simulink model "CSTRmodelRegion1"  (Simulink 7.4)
settings: Solver=ode15s  StartTime=0.0  StopTime=500  RelTol=1e-3
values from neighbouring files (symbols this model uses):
  cain = 2    [runDynSim321.m]    (also in sf_CSTR.m = cInVec(1))
  cbin = 1.5    [runDynSim321.m]    (also in sf_CSTR.m = cInVec(2))
undefined symbols (not defined in the file or in its folder): clamping, Floor, Ideal, internal, PI, sigbuilder_block
libraries: simulink_extras x2

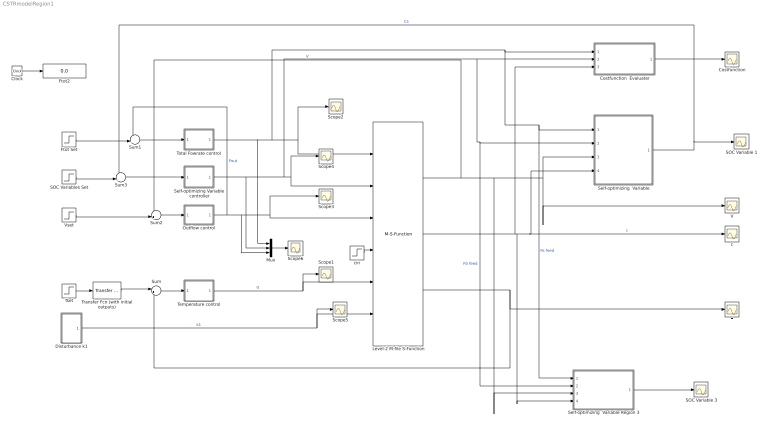
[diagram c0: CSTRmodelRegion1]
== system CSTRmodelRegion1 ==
  Clock : Clock
  Costfunction : Scope
  Costfunction  Evaluater : Subsystem
  Disturbance k1 : Subsystem
  Ftot Set : Step  Time=0  Before=22  After=22  SampleTime=0
  Ftot2 : Display
  Level-2 M-file S-Function : M-S-Function  FunctionName=sf_CSTR
  Mux : Mux  Inputs=3
  Outflow control : Subsystem  AncestorBlock=simulink/Continuous/PID Controller  DialogController=pidpack.PIDConfig.pidDDGCreate  DialogControllerArgs=DataTag2  mask(PID 1dof){Controller=PI, TimeDomain=Continuous-time, SampleTime=1, IntegratorMethod=Forward Euler, FilterMethod=Forward Euler, Form=Ideal, P=-5, I=0.8, D=0, N=100, InitialConditionSource=internal, InitialConditionForIntegrator=0, InitialConditionForFilter=0, ExternalReset=none, IgnoreLimit=off, ZeroCross=on, LimitOutput=off, UpperSaturationLimit=inf, LowerSaturationLimit=-inf, LinearizeAsGain=off, AntiWindupMode=none, Kb=1, TrackingMode=off, Kt=1, RndMeth=Floor, SaturateOnIntegerOverflow=off, LockScale=off, PParamMin=[], PParamMax=[], PParamDataTypeStr=Inherit: Inherit via internal rule, IParamMin=[], IParamMax=[], IParamDataTypeStr=Inherit: Inherit via internal rule, DParamMin=[], DParamMax=[], DParamDataTypeStr=Inherit: Inherit via internal rule, NParamMin=[], NParamMax=[], NParamDataTypeStr=Inherit: Inherit via internal rule, KbParamMin=[], KbParamMax=[], KbParamDataTypeStr=Inherit: Inherit via internal rule, KtParamMin=[], KtParamMax=[], KtParamDataTypeStr=Inherit: Inherit via internal rule, POutMin=[], POutMax=[], POutDataTypeStr=Inherit: Inherit via internal rule, IOutMin=[], IOutMax=[], IOutDataTypeStr=Inherit: Inherit via internal rule, DOutMin=[], DOutMax=[], DOutDataTypeStr=Inherit: Inherit via internal rule, NOutMin=[], NOutMax=[], NOutDataTypeStr=Inherit: Inherit via internal rule, KbOutMin=[], KbOutMax=[], KbOutDataTypeStr=Inherit: Inherit via internal rule, KtOutMin=[], KtOutMax=[], KtOutDataTypeStr=Inherit: Inherit via internal rule, IntegratorOutMin=[], IntegratorOutMax=[], IntegratorOutDataTypeStr=Inherit: Inherit via internal rule, FilterOutMin=[], FilterOutMax=[], FilterOutDataTypeStr=Inherit: Inherit via internal rule, SumOutMin=[], SumOutMax=[], SumOutDataTypeStr=Inherit: Inherit via internal rule, SumI1OutMin=[], SumI1OutMax=[], SumI1OutDataTypeStr=Inherit: Inherit via internal rule, SumI2OutMin=[], SumI2OutMax=[], SumI2OutDataTypeStr=Inherit: Inherit via internal rule, SumI3OutMin=[], SumI3OutMax=[], SumI3OutDataTypeStr=Inherit: Inherit via internal rule, SumDOutMin=[], SumDOutMax=[], SumDOutDataTypeStr=Inherit: Inherit via internal rule, SumAccumDataTypeStr=Inherit: Inherit via internal rule, SumI1AccumDataTypeStr=Inherit: Inherit via internal rule, SumI2AccumDataTypeStr=Inherit: Inherit via internal rule, SumI3AccumDataTypeStr=Inherit: Inherit via internal rule, SumDAccumDataTypeStr=Inherit: Inherit via internal rule, SaturationOutMin=[], SaturationOutMax=[], SaturationOutDataTypeStr=Inherit: Same as input, IntegratorContinuousStateAttributes='', IntegratorStateIdentifier=, IntegratorStateMustResolveToSignalObject=off, IntegratorRTWStateStorageClass=Auto, IntegratorRTWStateStorageTypeQualifier=, FilterContinuousStateAttributes='', FilterStateIdentifier=, FilterStateMustResolveToSignalObject=off, FilterRTWStateStorageClass=Auto, FilterRTWStateStorageTypeQualifier=}
      mask prompts: TimeDomain "Time-domain:"; SampleTime "Sample time (-1 for inherited):"; IntegratorMethod "Integrator method:"; FilterMethod "Filter method:"; Form "Controller form:"; P "Proportional (P):"; I "Integral (I):"; D "Derivative (D):"; N "Filter coefficient (N):"; InitialConditionSource "Source:"; InitialConditionForIntegrator "Integrator:"; InitialConditionForFilter "Filter:"; ExternalReset "External reset:"; IgnoreLimit "Ignore reset when linearizing"; ZeroCross "Enable zero-crossing detection"; LimitOutput "Limit output"; UpperSaturationLimit "Upper saturation limit:"; LowerSaturationLimit "Lower saturation limit:"; LinearizeAsGain "Ignore saturation when linearizing"; AntiWindupMode "Anti-windup method:"; Kb "Back-calculation coefficient (Kb):"; TrackingMode "Enable tracking mode"; Kt "Tracking coefficient (Kt):"; RndMeth "Integer rounding mode:"; SaturateOnIntegerOverflow "Saturate on integer overflow"; LockScale "Lock data type settings against changes by the fixed-point tools"; PParamMin "P parameter minimum:"; PParamMax "P parameter maximum:"; PParamDataTypeStr "P parameter:"; IParamMin "I parameter minimum:"; IParamMax "I parameter maximum:"; IParamDataTypeStr "I parameter:"; DParamMin "D parameter minimum:"; DParamMax "D parameter maximum:"; DParamDataTypeStr "D parameter:"; NParamMin "N parameter minimum:"; NParamMax "N parameter maximum:"; NParamDataTypeStr "N parameter:"; KbParamMin "Kb parameter minimum:"; KbParamMax "Kb parameter maximum:"; KbParamDataTypeStr "Kb parameter:"; KtParamMin "Kt parameter minimum:"; KtParamMax "Kt parameter maximum:"; KtParamDataTypeStr "Kt parameter:"; POutMin "P product output minimum:"; POutMax "P product output maximum:"; POutDataTypeStr "P product output:"; IOutMin "I product output minimum:"; IOutMax "I product output maximum:"; IOutDataTypeStr "I product output:"; DOutMin "D product output minimum:"; DOutMax "D product output maximum:"; DOutDataTypeStr "D product output:"; NOutMin "N product output minimum:"; NOutMax "N product output maximum:"; NOutDataTypeStr "N product output:"; KbOutMin "Kb product output minimum:"; KbOutMax "Kb product output maximum:"; KbOutDataTypeStr "Kb product output:"; KtOutMin "Kt product output minimum:"; KtOutMax "Kt product output maximum:"; KtOutDataTypeStr "Kt product output:"; IntegratorOutMin "Integrator output minimum:"; IntegratorOutMax "Integrator output maximum:"; IntegratorOutDataTypeStr "Integrator output:"; FilterOutMin "Filter output minimum:"; FilterOutMax "Filter output maximum:"; FilterOutDataTypeStr "Filter output:"; SumOutMin "Sum output minimum:"; SumOutMax "Sum output maximum:"; SumOutDataTypeStr "Sum output:"; SumI1OutMin "SumI1 output minimum:"; SumI1OutMax "SumI1 output maximum:"; SumI1OutDataTypeStr "SumI1 output:"; SumI2OutMin "SumI2 output minimum:"; SumI2OutMax "SumI2 output maximum:"; SumI2OutDataTypeStr "SumI2 output:"; SumI3OutMin "SumI3 output minimum:"; SumI3OutMax "SumI3 output maximum:"; SumI3OutDataTypeStr "SumI3 output:"; SumDOutMin "SumD output minimum:"; SumDOutMax "SumD output maximum:"; SumDOutDataTypeStr "SumD output:"; SumAccumDataTypeStr "Accumulator of Sum:"; SumI1AccumDataTypeStr "Accumulator of SumI1:"; SumI2AccumDataTypeStr "Accumulator of SumI2:"; SumI3AccumDataTypeStr "Accumulator of SumI3:"; SumDAccumDataTypeStr "Accumulator of SumD:"; SaturationOutMin "Saturation output minimum:"; SaturationOutMax "Saturation output maximum:"; SaturationOutDataTypeStr "Saturation output:"; IntegratorContinuousStateAttributes "State name: (e.g., 'position')"; IntegratorStateIdentifier "State name:"; IntegratorStateMustResolveToSignalObject "State name must resolve to Simulink signal object"; IntegratorRTWStateStorageClass "Real-Time Workshop storage class:"; IntegratorRTWStateStorageTypeQualifier "Real-Time Workshop storage type qualifier:"; FilterContinuousStateAttributes "State name: (e.g., 'position')"; FilterStateIdentifier "State name:"; FilterStateMustResolveToSignalObject "State name must resolve to Simulink signal object"; FilterRTWStateStorageClass "Real-Time Workshop storage class:"; FilterRTWStateStorageTypeQualifier "Real-Time Workshop storage type qualifier:"
      mask help: This block implements continuous- and discrete-time PID control algorithms and includes advanced features such as anti-windup, external reset, and signal tracking. You can tune the PID gains automatically using the 'Tune...' button (requires Simulink Control Design).
      mask init:
      | [shiftx shifty satshiftx satshifty] = pidpack.PIDConfig.configPID(gcbh);
  SOC Variable 1 : Scope
  SOC Variable 3 : Scope
  SOC Variables Set : Step  Time=0  After=0  SampleTime=0
  Scope{1..6} (6 alike) : Scope
  Self-optimizing  Variable : Stateflow chart
  Self-optimizing  Variable Region 3 : Stateflow chart
  Self-optimizing Variable  controller : Subsystem  AncestorBlock=simulink/Continuous/PID Controller  DialogController=pidpack.PIDConfig.pidDDGCreate  DialogControllerArgs=DataTag3  mask(PID 1dof){Controller=PI, TimeDomain=Continuous-time, SampleTime=1, IntegratorMethod=Forward Euler, FilterMethod=Forward Euler, Form=Ideal, P=145, I=3, D=0, N=100, InitialConditionSource=internal, InitialConditionForIntegrator=0, InitialConditionForFilter=0, ExternalReset=none, IgnoreLimit=off, ZeroCross=on, LimitOutput=off, UpperSaturationLimit=1e6, LowerSaturationLimit=0, LinearizeAsGain=off, AntiWindupMode=none, Kb=1, TrackingMode=off, Kt=1, RndMeth=Floor, SaturateOnIntegerOverflow=off, LockScale=off, PParamMin=[], PParamMax=[], PParamDataTypeStr=Inherit: Inherit via internal rule, IParamMin=[], IParamMax=[], IParamDataTypeStr=Inherit: Inherit via internal rule, DParamMin=[], DParamMax=[], DParamDataTypeStr=Inherit: Inherit via internal rule, NParamMin=[], NParamMax=[], NParamDataTypeStr=Inherit: Inherit via internal rule, KbParamMin=[], KbParamMax=[], KbParamDataTypeStr=Inherit: Inherit via internal rule, KtParamMin=[], KtParamMax=[], KtParamDataTypeStr=Inherit: Inherit via internal rule, POutMin=[], POutMax=[], POutDataTypeStr=Inherit: Inherit via internal rule, IOutMin=[], IOutMax=[], IOutDataTypeStr=Inherit: Inherit via internal rule, DOutMin=[], DOutMax=[], DOutDataTypeStr=Inherit: Inherit via internal rule, NOutMin=[], NOutMax=[], NOutDataTypeStr=Inherit: Inherit via internal rule, KbOutMin=[], KbOutMax=[], KbOutDataTypeStr=Inherit: Inherit via internal rule, KtOutMin=[], KtOutMax=[], KtOutDataTypeStr=Inherit: Inherit via internal rule, IntegratorOutMin=[], IntegratorOutMax=[], IntegratorOutDataTypeStr=Inherit: Inherit via internal rule, FilterOutMin=[], FilterOutMax=[], FilterOutDataTypeStr=Inherit: Inherit via internal rule, SumOutMin=[], SumOutMax=[], SumOutDataTypeStr=Inherit: Inherit via internal rule, SumI1OutMin=[], SumI1OutMax=[], SumI1OutDataTypeStr=Inherit: Inherit via internal rule, SumI2OutMin=[], SumI2OutMax=[], SumI2OutDataTypeStr=Inherit: Inherit via internal rule, SumI3OutMin=[], SumI3OutMax=[], SumI3OutDataTypeStr=Inherit: Inherit via internal rule, SumDOutMin=[], SumDOutMax=[], SumDOutDataTypeStr=Inherit: Inherit via internal rule, SumAccumDataTypeStr=Inherit: Inherit via internal rule, SumI1AccumDataTypeStr=Inherit: Inherit via internal rule, SumI2AccumDataTypeStr=Inherit: Inherit via internal rule, SumI3AccumDataTypeStr=Inherit: Inherit via internal rule, SumDAccumDataTypeStr=Inherit: Inherit via internal rule, SaturationOutMin=[], SaturationOutMax=[], SaturationOutDataTypeStr=Inherit: Same as input, IntegratorContinuousStateAttributes='', IntegratorStateIdentifier=, IntegratorStateMustResolveToSignalObject=off, IntegratorRTWStateStorageClass=Auto, IntegratorRTWStateStorageTypeQualifier=, FilterContinuousStateAttributes='', FilterStateIdentifier=, FilterStateMustResolveToSignalObject=off, FilterRTWStateStorageClass=Auto, FilterRTWStateStorageTypeQualifier=}
      mask prompts: TimeDomain "Time-domain:"; SampleTime "Sample time (-1 for inherited):"; IntegratorMethod "Integrator method:"; FilterMethod "Filter method:"; Form "Controller form:"; P "Proportional (P):"; I "Integral (I):"; D "Derivative (D):"; N "Filter coefficient (N):"; InitialConditionSource "Source:"; InitialConditionForIntegrator "Integrator:"; InitialConditionForFilter "Filter:"; ExternalReset "External reset:"; IgnoreLimit "Ignore reset when linearizing"; ZeroCross "Enable zero-crossing detection"; LimitOutput "Limit output"; UpperSaturationLimit "Upper saturation limit:"; LowerSaturationLimit "Lower saturation limit:"; LinearizeAsGain "Ignore saturation when linearizing"; AntiWindupMode "Anti-windup method:"; Kb "Back-calculation coefficient (Kb):"; TrackingMode "Enable tracking mode"; Kt "Tracking coefficient (Kt):"; RndMeth "Integer rounding mode:"; SaturateOnIntegerOverflow "Saturate on integer overflow"; LockScale "Lock data type settings against changes by the fixed-point tools"; PParamMin "P parameter minimum:"; PParamMax "P parameter maximum:"; PParamDataTypeStr "P parameter:"; IParamMin "I parameter minimum:"; IParamMax "I parameter maximum:"; IParamDataTypeStr "I parameter:"; DParamMin "D parameter minimum:"; DParamMax "D parameter maximum:"; DParamDataTypeStr "D parameter:"; NParamMin "N parameter minimum:"; NParamMax "N parameter maximum:"; NParamDataTypeStr "N parameter:"; KbParamMin "Kb parameter minimum:"; KbParamMax "Kb parameter maximum:"; KbParamDataTypeStr "Kb parameter:"; KtParamMin "Kt parameter minimum:"; KtParamMax "Kt parameter maximum:"; KtParamDataTypeStr "Kt parameter:"; POutMin "P product output minimum:"; POutMax "P product output maximum:"; POutDataTypeStr "P product output:"; IOutMin "I product output minimum:"; IOutMax "I product output maximum:"; IOutDataTypeStr "I product output:"; DOutMin "D product output minimum:"; DOutMax "D product output maximum:"; DOutDataTypeStr "D product output:"; NOutMin "N product output minimum:"; NOutMax "N product output maximum:"; NOutDataTypeStr "N product output:"; KbOutMin "Kb product output minimum:"; KbOutMax "Kb product output maximum:"; KbOutDataTypeStr "Kb product output:"; KtOutMin "Kt product output minimum:"; KtOutMax "Kt product output maximum:"; KtOutDataTypeStr "Kt product output:"; IntegratorOutMin "Integrator output minimum:"; IntegratorOutMax "Integrator output maximum:"; IntegratorOutDataTypeStr "Integrator output:"; FilterOutMin "Filter output minimum:"; FilterOutMax "Filter output maximum:"; FilterOutDataTypeStr "Filter output:"; SumOutMin "Sum output minimum:"; SumOutMax "Sum output maximum:"; SumOutDataTypeStr "Sum output:"; SumI1OutMin "SumI1 output minimum:"; SumI1OutMax "SumI1 output maximum:"; SumI1OutDataTypeStr "SumI1 output:"; SumI2OutMin "SumI2 output minimum:"; SumI2OutMax "SumI2 output maximum:"; SumI2OutDataTypeStr "SumI2 output:"; SumI3OutMin "SumI3 output minimum:"; SumI3OutMax "SumI3 output maximum:"; SumI3OutDataTypeStr "SumI3 output:"; SumDOutMin "SumD output minimum:"; SumDOutMax "SumD output maximum:"; SumDOutDataTypeStr "SumD output:"; SumAccumDataTypeStr "Accumulator of Sum:"; SumI1AccumDataTypeStr "Accumulator of SumI1:"; SumI2AccumDataTypeStr "Accumulator of SumI2:"; SumI3AccumDataTypeStr "Accumulator of SumI3:"; SumDAccumDataTypeStr "Accumulator of SumD:"; SaturationOutMin "Saturation output minimum:"; SaturationOutMax "Saturation output maximum:"; SaturationOutDataTypeStr "Saturation output:"; IntegratorContinuousStateAttributes "State name: (e.g., 'position')"; IntegratorStateIdentifier "State name:"; IntegratorStateMustResolveToSignalObject "State name must resolve to Simulink signal object"; IntegratorRTWStateStorageClass "Real-Time Workshop storage class:"; IntegratorRTWStateStorageTypeQualifier "Real-Time Workshop storage type qualifier:"; FilterContinuousStateAttributes "State name: (e.g., 'position')"; FilterStateIdentifier "State name:"; FilterStateMustResolveToSignalObject "State name must resolve to Simulink signal object"; FilterRTWStateStorageClass "Real-Time Workshop storage class:"; FilterRTWStateStorageTypeQualifier "Real-Time Workshop storage type qualifier:"
      mask help: This block implements continuous- and discrete-time PID control algorithms and includes advanced features such as anti-windup, external reset, and signal tracking. You can tune the PID gains automatically using the 'Tune...' button (requires Simulink Control Design).
      mask init:
      | [shiftx shifty satshiftx satshifty] = pidpack.PIDConfig.configPID(gcbh);
  Sum : Sum  Inputs=|+-  OutDataType=fixdt(1, 16)  OutScaling=2^0
  Sum1 : Sum  Inputs=-+|  OutDataType=fixdt(1, 16)  OutScaling=2^0
  Sum2 : Sum  Inputs=-+|  OutDataType=fixdt(1, 16)  OutScaling=2^0
  Sum3 : Sum  Inputs=-+|  OutDataType=fixdt(1, 16)  OutScaling=2^0
  T : Scope
  Temperature control : Subsystem  AncestorBlock=simulink/Continuous/PID Controller  DialogController=pidpack.PIDConfig.pidDDGCreate  DialogControllerArgs=DataTag4  mask(PID 1dof){Controller=PI, TimeDomain=Continuous-time, SampleTime=1, IntegratorMethod=Forward Euler, FilterMethod=Forward Euler, Form=Ideal, P=-3521, I=2.4, D=0, N=100, InitialConditionSource=internal, InitialConditionForIntegrator=888, InitialConditionForFilter=0, ExternalReset=none, IgnoreLimit=off, ZeroCross=on, LimitOutput=on, UpperSaturationLimit=1e3, LowerSaturationLimit=0, LinearizeAsGain=off, AntiWindupMode=clamping, Kb=1, TrackingMode=off, Kt=1, RndMeth=Floor, SaturateOnIntegerOverflow=off, LockScale=off, PParamMin=[], PParamMax=[], PParamDataTypeStr=Inherit: Inherit via internal rule, IParamMin=[], IParamMax=[], IParamDataTypeStr=Inherit: Inherit via internal rule, DParamMin=[], DParamMax=[], DParamDataTypeStr=Inherit: Inherit via internal rule, NParamMin=[], NParamMax=[], NParamDataTypeStr=Inherit: Inherit via internal rule, KbParamMin=[], KbParamMax=[], KbParamDataTypeStr=Inherit: Inherit via internal rule, KtParamMin=[], KtParamMax=[], KtParamDataTypeStr=Inherit: Inherit via internal rule, POutMin=[], POutMax=[], POutDataTypeStr=Inherit: Inherit via internal rule, IOutMin=[], IOutMax=[], IOutDataTypeStr=Inherit: Inherit via internal rule, DOutMin=[], DOutMax=[], DOutDataTypeStr=Inherit: Inherit via internal rule, NOutMin=[], NOutMax=[], NOutDataTypeStr=Inherit: Inherit via internal rule, KbOutMin=[], KbOutMax=[], KbOutDataTypeStr=Inherit: Inherit via internal rule, KtOutMin=[], KtOutMax=[], KtOutDataTypeStr=Inherit: Inherit via internal rule, IntegratorOutMin=[], IntegratorOutMax=[], IntegratorOutDataTypeStr=Inherit: Inherit via internal rule, FilterOutMin=[], FilterOutMax=[], FilterOutDataTypeStr=Inherit: Inherit via internal rule, SumOutMin=[], SumOutMax=[], SumOutDataTypeStr=Inherit: Inherit via internal rule, SumI1OutMin=[], SumI1OutMax=[], SumI1OutDataTypeStr=Inherit: Inherit via internal rule, SumI2OutMin=[], SumI2OutMax=[], SumI2OutDataTypeStr=Inherit: Inherit via internal rule, SumI3OutMin=[], SumI3OutMax=[], SumI3OutDataTypeStr=Inherit: Inherit via internal rule, SumDOutMin=[], SumDOutMax=[], SumDOutDataTypeStr=Inherit: Inherit via internal rule, SumAccumDataTypeStr=Inherit: Inherit via internal rule, SumI1AccumDataTypeStr=Inherit: Inherit via internal rule, SumI2AccumDataTypeStr=Inherit: Inherit via internal rule, SumI3AccumDataTypeStr=Inherit: Inherit via internal rule, SumDAccumDataTypeStr=Inherit: Inherit via internal rule, SaturationOutMin=[], SaturationOutMax=[], SaturationOutDataTypeStr=Inherit: Same as input, IntegratorContinuousStateAttributes='', IntegratorStateIdentifier=, IntegratorStateMustResolveToSignalObject=off, IntegratorRTWStateStorageClass=Auto, IntegratorRTWStateStorageTypeQualifier=, FilterContinuousStateAttributes='', FilterStateIdentifier=, FilterStateMustResolveToSignalObject=off, FilterRTWStateStorageClass=Auto, FilterRTWStateStorageTypeQualifier=}
      mask prompts: TimeDomain "Time-domain:"; SampleTime "Sample time (-1 for inherited):"; IntegratorMethod "Integrator method:"; FilterMethod "Filter method:"; Form "Controller form:"; P "Proportional (P):"; I "Integral (I):"; D "Derivative (D):"; N "Filter coefficient (N):"; InitialConditionSource "Source:"; InitialConditionForIntegrator "Integrator:"; InitialConditionForFilter "Filter:"; ExternalReset "External reset:"; IgnoreLimit "Ignore reset when linearizing"; ZeroCross "Enable zero-crossing detection"; LimitOutput "Limit output"; UpperSaturationLimit "Upper saturation limit:"; LowerSaturationLimit "Lower saturation limit:"; LinearizeAsGain "Ignore saturation when linearizing"; AntiWindupMode "Anti-windup method:"; Kb "Back-calculation coefficient (Kb):"; TrackingMode "Enable tracking mode"; Kt "Tracking coefficient (Kt):"; RndMeth "Integer rounding mode:"; SaturateOnIntegerOverflow "Saturate on integer overflow"; LockScale "Lock data type settings against changes by the fixed-point tools"; PParamMin "P parameter minimum:"; PParamMax "P parameter maximum:"; PParamDataTypeStr "P parameter:"; IParamMin "I parameter minimum:"; IParamMax "I parameter maximum:"; IParamDataTypeStr "I parameter:"; DParamMin "D parameter minimum:"; DParamMax "D parameter maximum:"; DParamDataTypeStr "D parameter:"; NParamMin "N parameter minimum:"; NParamMax "N parameter maximum:"; NParamDataTypeStr "N parameter:"; KbParamMin "Kb parameter minimum:"; KbParamMax "Kb parameter maximum:"; KbParamDataTypeStr "Kb parameter:"; KtParamMin "Kt parameter minimum:"; KtParamMax "Kt parameter maximum:"; KtParamDataTypeStr "Kt parameter:"; POutMin "P product output minimum:"; POutMax "P product output maximum:"; POutDataTypeStr "P product output:"; IOutMin "I product output minimum:"; IOutMax "I product output maximum:"; IOutDataTypeStr "I product output:"; DOutMin "D product output minimum:"; DOutMax "D product output maximum:"; DOutDataTypeStr "D product output:"; NOutMin "N product output minimum:"; NOutMax "N product output maximum:"; NOutDataTypeStr "N product output:"; KbOutMin "Kb product output minimum:"; KbOutMax "Kb product output maximum:"; KbOutDataTypeStr "Kb product output:"; KtOutMin "Kt product output minimum:"; KtOutMax "Kt product output maximum:"; KtOutDataTypeStr "Kt product output:"; IntegratorOutMin "Integrator output minimum:"; IntegratorOutMax "Integrator output maximum:"; IntegratorOutDataTypeStr "Integrator output:"; FilterOutMin "Filter output minimum:"; FilterOutMax "Filter output maximum:"; FilterOutDataTypeStr "Filter output:"; SumOutMin "Sum output minimum:"; SumOutMax "Sum output maximum:"; SumOutDataTypeStr "Sum output:"; SumI1OutMin "SumI1 output minimum:"; SumI1OutMax "SumI1 output maximum:"; SumI1OutDataTypeStr "SumI1 output:"; SumI2OutMin "SumI2 output minimum:"; SumI2OutMax "SumI2 output maximum:"; SumI2OutDataTypeStr "SumI2 output:"; SumI3OutMin "SumI3 output minimum:"; SumI3OutMax "SumI3 output maximum:"; SumI3OutDataTypeStr "SumI3 output:"; SumDOutMin "SumD output minimum:"; SumDOutMax "SumD output maximum:"; SumDOutDataTypeStr "SumD output:"; SumAccumDataTypeStr "Accumulator of Sum:"; SumI1AccumDataTypeStr "Accumulator of SumI1:"; SumI2AccumDataTypeStr "Accumulator of SumI2:"; SumI3AccumDataTypeStr "Accumulator of SumI3:"; SumDAccumDataTypeStr "Accumulator of SumD:"; SaturationOutMin "Saturation output minimum:"; SaturationOutMax "Saturation output maximum:"; SaturationOutDataTypeStr "Saturation output:"; IntegratorContinuousStateAttributes "State name: (e.g., 'position')"; IntegratorStateIdentifier "State name:"; IntegratorStateMustResolveToSignalObject "State name must resolve to Simulink signal object"; IntegratorRTWStateStorageClass "Real-Time Workshop storage class:"; IntegratorRTWStateStorageTypeQualifier "Real-Time Workshop storage type qualifier:"; FilterContinuousStateAttributes "State name: (e.g., 'position')"; FilterStateIdentifier "State name:"; FilterStateMustResolveToSignalObject "State name must resolve to Simulink signal object"; FilterRTWStateStorageClass "Real-Time Workshop storage class:"; FilterRTWStateStorageTypeQualifier "Real-Time Workshop storage type qualifier:"
      mask help: This block implements continuous- and discrete-time PID control algorithms and includes advanced features such as anti-windup, external reset, and signal tracking. You can tune the PID gains automatically using the 'Tune...' button (requires Simulink Control Design).
      mask init:
      | [shiftx shifty satshiftx satshifty] = pidpack.PIDConfig.configPID(gcbh);
  Total Fowrate control : Subsystem  AncestorBlock=simulink/Continuous/PID Controller  DialogController=pidpack.PIDConfig.pidDDGCreate  DialogControllerArgs=DataTag5  mask(PID 1dof){Controller=PI, TimeDomain=Continuous-time, SampleTime=1, IntegratorMethod=Forward Euler, FilterMethod=Forward Euler, Form=Ideal, P=0.58, I=0.35, D=0, N=100, InitialConditionSource=internal, InitialConditionForIntegrator=0, InitialConditionForFilter=0, ExternalReset=none, IgnoreLimit=off, ZeroCross=on, LimitOutput=off, UpperSaturationLimit=1e6, LowerSaturationLimit=0, LinearizeAsGain=off, AntiWindupMode=none, Kb=1, TrackingMode=off, Kt=1, RndMeth=Floor, SaturateOnIntegerOverflow=off, LockScale=off, PParamMin=[], PParamMax=[], PParamDataTypeStr=Inherit: Inherit via internal rule, IParamMin=[], IParamMax=[], IParamDataTypeStr=Inherit: Inherit via internal rule, DParamMin=[], DParamMax=[], DParamDataTypeStr=Inherit: Inherit via internal rule, NParamMin=[], NParamMax=[], NParamDataTypeStr=Inherit: Inherit via internal rule, KbParamMin=[], KbParamMax=[], KbParamDataTypeStr=Inherit: Inherit via internal rule, KtParamMin=[], KtParamMax=[], KtParamDataTypeStr=Inherit: Inherit via internal rule, POutMin=[], POutMax=[], POutDataTypeStr=Inherit: Inherit via internal rule, IOutMin=[], IOutMax=[], IOutDataTypeStr=Inherit: Inherit via internal rule, DOutMin=[], DOutMax=[], DOutDataTypeStr=Inherit: Inherit via internal rule, NOutMin=[], NOutMax=[], NOutDataTypeStr=Inherit: Inherit via internal rule, KbOutMin=[], KbOutMax=[], KbOutDataTypeStr=Inherit: Inherit via internal rule, KtOutMin=[], KtOutMax=[], KtOutDataTypeStr=Inherit: Inherit via internal rule, IntegratorOutMin=[], IntegratorOutMax=[], IntegratorOutDataTypeStr=Inherit: Inherit via internal rule, FilterOutMin=[], FilterOutMax=[], FilterOutDataTypeStr=Inherit: Inherit via internal rule, SumOutMin=[], SumOutMax=[], SumOutDataTypeStr=Inherit: Inherit via internal rule, SumI1OutMin=[], SumI1OutMax=[], SumI1OutDataTypeStr=Inherit: Inherit via internal rule, SumI2OutMin=[], SumI2OutMax=[], SumI2OutDataTypeStr=Inherit: Inherit via internal rule, SumI3OutMin=[], SumI3OutMax=[], SumI3OutDataTypeStr=Inherit: Inherit via internal rule, SumDOutMin=[], SumDOutMax=[], SumDOutDataTypeStr=Inherit: Inherit via internal rule, SumAccumDataTypeStr=Inherit: Inherit via internal rule, SumI1AccumDataTypeStr=Inherit: Inherit via internal rule, SumI2AccumDataTypeStr=Inherit: Inherit via internal rule, SumI3AccumDataTypeStr=Inherit: Inherit via internal rule, SumDAccumDataTypeStr=Inherit: Inherit via internal rule, SaturationOutMin=[], SaturationOutMax=[], SaturationOutDataTypeStr=Inherit: Same as input, IntegratorContinuousStateAttributes='', IntegratorStateIdentifier=, IntegratorStateMustResolveToSignalObject=off, IntegratorRTWStateStorageClass=Auto, IntegratorRTWStateStorageTypeQualifier=, FilterContinuousStateAttributes='', FilterStateIdentifier=, FilterStateMustResolveToSignalObject=off, FilterRTWStateStorageClass=Auto, FilterRTWStateStorageTypeQualifier=}
      mask prompts: TimeDomain "Time-domain:"; SampleTime "Sample time (-1 for inherited):"; IntegratorMethod "Integrator method:"; FilterMethod "Filter method:"; Form "Controller form:"; P "Proportional (P):"; I "Integral (I):"; D "Derivative (D):"; N "Filter coefficient (N):"; InitialConditionSource "Source:"; InitialConditionForIntegrator "Integrator:"; InitialConditionForFilter "Filter:"; ExternalReset "External reset:"; IgnoreLimit "Ignore reset when linearizing"; ZeroCross "Enable zero-crossing detection"; LimitOutput "Limit output"; UpperSaturationLimit "Upper saturation limit:"; LowerSaturationLimit "Lower saturation limit:"; LinearizeAsGain "Ignore saturation when linearizing"; AntiWindupMode "Anti-windup method:"; Kb "Back-calculation coefficient (Kb):"; TrackingMode "Enable tracking mode"; Kt "Tracking coefficient (Kt):"; RndMeth "Integer rounding mode:"; SaturateOnIntegerOverflow "Saturate on integer overflow"; LockScale "Lock data type settings against changes by the fixed-point tools"; PParamMin "P parameter minimum:"; PParamMax "P parameter maximum:"; PParamDataTypeStr "P parameter:"; IParamMin "I parameter minimum:"; IParamMax "I parameter maximum:"; IParamDataTypeStr "I parameter:"; DParamMin "D parameter minimum:"; DParamMax "D parameter maximum:"; DParamDataTypeStr "D parameter:"; NParamMin "N parameter minimum:"; NParamMax "N parameter maximum:"; NParamDataTypeStr "N parameter:"; KbParamMin "Kb parameter minimum:"; KbParamMax "Kb parameter maximum:"; KbParamDataTypeStr "Kb parameter:"; KtParamMin "Kt parameter minimum:"; KtParamMax "Kt parameter maximum:"; KtParamDataTypeStr "Kt parameter:"; POutMin "P product output minimum:"; POutMax "P product output maximum:"; POutDataTypeStr "P product output:"; IOutMin "I product output minimum:"; IOutMax "I product output maximum:"; IOutDataTypeStr "I product output:"; DOutMin "D product output minimum:"; DOutMax "D product output maximum:"; DOutDataTypeStr "D product output:"; NOutMin "N product output minimum:"; NOutMax "N product output maximum:"; NOutDataTypeStr "N product output:"; KbOutMin "Kb product output minimum:"; KbOutMax "Kb product output maximum:"; KbOutDataTypeStr "Kb product output:"; KtOutMin "Kt product output minimum:"; KtOutMax "Kt product output maximum:"; KtOutDataTypeStr "Kt product output:"; IntegratorOutMin "Integrator output minimum:"; IntegratorOutMax "Integrator output maximum:"; IntegratorOutDataTypeStr "Integrator output:"; FilterOutMin "Filter output minimum:"; FilterOutMax "Filter output maximum:"; FilterOutDataTypeStr "Filter output:"; SumOutMin "Sum output minimum:"; SumOutMax "Sum output maximum:"; SumOutDataTypeStr "Sum output:"; SumI1OutMin "SumI1 output minimum:"; SumI1OutMax "SumI1 output maximum:"; SumI1OutDataTypeStr "SumI1 output:"; SumI2OutMin "SumI2 output minimum:"; SumI2OutMax "SumI2 output maximum:"; SumI2OutDataTypeStr "SumI2 output:"; SumI3OutMin "SumI3 output minimum:"; SumI3OutMax "SumI3 output maximum:"; SumI3OutDataTypeStr "SumI3 output:"; SumDOutMin "SumD output minimum:"; SumDOutMax "SumD output maximum:"; SumDOutDataTypeStr "SumD output:"; SumAccumDataTypeStr "Accumulator of Sum:"; SumI1AccumDataTypeStr "Accumulator of SumI1:"; SumI2AccumDataTypeStr "Accumulator of SumI2:"; SumI3AccumDataTypeStr "Accumulator of SumI3:"; SumDAccumDataTypeStr "Accumulator of SumD:"; SaturationOutMin "Saturation output minimum:"; SaturationOutMax "Saturation output maximum:"; SaturationOutDataTypeStr "Saturation output:"; IntegratorContinuousStateAttributes "State name: (e.g., 'position')"; IntegratorStateIdentifier "State name:"; IntegratorStateMustResolveToSignalObject "State name must resolve to Simulink signal object"; IntegratorRTWStateStorageClass "Real-Time Workshop storage class:"; IntegratorRTWStateStorageTypeQualifier "Real-Time Workshop storage type qualifier:"; FilterContinuousStateAttributes "State name: (e.g., 'position')"; FilterStateIdentifier "State name:"; FilterStateMustResolveToSignalObject "State name must resolve to Simulink signal object"; FilterRTWStateStorageClass "Real-Time Workshop storage class:"; FilterRTWStateStorageTypeQualifier "Real-Time Workshop storage type qualifier:"
      mask help: This block implements continuous- and discrete-time PID control algorithms and includes advanced features such as anti-windup, external reset, and signal tracking. You can tune the PID gains automatically using the 'Tune...' button (requires Simulink Control Design).
      mask init:
      | [shiftx shifty satshiftx satshifty] = pidpack.PIDConfig.configPID(gcbh);
  Transfer Fcn (with initial outputs) : simulink_extras/Additional Linear/Transfer Fcn (with initial outputs)  SystemSampleTime=-1  N=[1]  D="[10  1]"  Y0=350  U0=0
  Tset : Step  Time=250  Before=350  After=350  SampleTime=0
  V : Scope
  Vset : Step  Time=0  Before=500  After=500  SampleTime=0
  c : Scope
  cin : Step  Time=0  Before=[cain cbin 0 0]  After=[cain cbin 0 0]  SampleTime=0
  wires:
  cin/1 -> Level-2 M-file S-Function/4
  Sum/1 -> Temperature control/1(u)
  Level-2 M-file S-Function/1 -> Sum2/1, Self-optimizing  Variable/3(V), V/1, Self-optimizing  Variable Region 3/3(V)  "V"
  Level-2 M-file S-Function/2 -> Costfunction  Evaluater/3(Concentrations), c/1, Self-optimizing  Variable/4(cVector), Self-optimizing  Variable Region 3/4(cVector)  "c"
  Level-2 M-file S-Function/3 -> T/1, Sum/2  "T"
  Tset/1 -> Transfer Fcn (with initial outputs)/1
  Vset/1 -> Sum2/2
  Sum2/1 -> Outflow control/1(u)
  Costfunction  Evaluater/1(Objective) -> Costfunction/1
  Outflow control/1(y) -> Sum1/1, Level-2 M-file S-Function/3, Scope3/1, Mux/3  "Fout"
  Temperature control/1(y) -> Level-2 M-file S-Function/5, Scope1/1  "q"
  Sum1/1 -> Total Fowrate control/1(u)
  Total Fowrate control/1(y) -> Level-2 M-file S-Function/1, Scope2/1, Costfunction  Evaluater/1(Fa), Self-optimizing  Variable/1(Fa), Self-optimizing  Variable Region 3/1(Fa), Mux/1  "Fa feed"
  Self-optimizing  Variable/1(cs) -> Sum3/1, SOC Variable 1/1  "Cs"
  SOC Variables Set/1 -> Sum3/2
  Sum3/1 -> Self-optimizing Variable  controller/1(u)
  Self-optimizing Variable  controller/1(y) -> Level-2 M-file S-Function/2, Scope4/1, Costfunction  Evaluater/2(Fb), Self-optimizing  Variable Region 3/2(Fb), Self-optimizing  Variable/2(Fb), Mux/2  "Fb feed"
  Ftot Set/1 -> Sum1/2
  Disturbance k1/1(Out1) -> Level-2 M-file S-Function/6, Scope5/1  "k1"
  Transfer Fcn (with initial outputs)/1 -> Sum/1
  Mux/1 -> Scope6/1
  Clock/1 -> Ftot2/1
  Self-optimizing  Variable Region 3/1(cs) -> SOC Variable 3/1

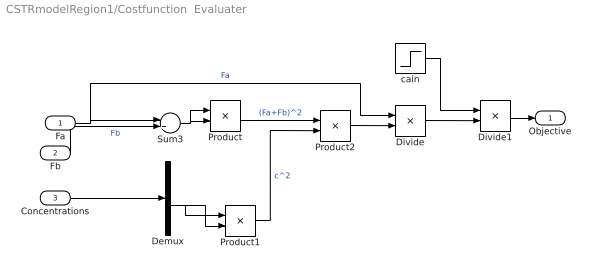
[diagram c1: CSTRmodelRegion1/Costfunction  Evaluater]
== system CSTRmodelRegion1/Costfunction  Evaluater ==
  Fa : Inport
  Fb : Inport  Port=2
  Concentrations : Inport  Port=3
  Demux : Demux
  Divide : Product  Inputs=/*  OutDataType=fixdt(1, 16)  OutScaling=2^-10
  Divide1 : Product  Inputs=/*  OutDataType=fixdt(1, 16)  OutScaling=2^-10
  Product : Product  OutDataType=fixdt(1, 16)  OutScaling=2^0
  Product1 : Product  OutDataType=fixdt(1, 16)  OutScaling=2^0
  Product2 : Product  OutDataType=fixdt(1, 16)  OutScaling=2^0
  Sum3 : Sum  Inputs=|++  OutDataType=fixdt(1, 16)  OutScaling=2^0
  cain : Step  Before=cain  After=cain  SampleTime=0
  Objective : Outport
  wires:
  Sum3/1 -> Product/1, Product/2
  Demux/3 -> Product1/2, Product1/1
  Product/1 -> Product2/1  "(Fa+Fb)^2"
  Product1/1 -> Product2/2  "c^2"
  Product2/1 -> Divide/2
  Divide/1 -> Divide1/2
  cain/1 -> Divide1/1
  Fa/1 -> Sum3/1, Divide/1  "Fa"
  Fb/1 -> Sum3/2  "Fb"
  Concentrations/1 -> Demux/1
  Divide1/1 -> Objective/1
  Demux/1 -> ?
  Demux/2 -> ?
  Demux/4 -> ?

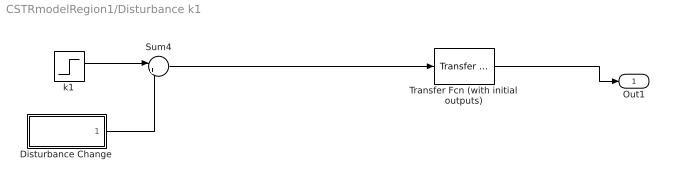
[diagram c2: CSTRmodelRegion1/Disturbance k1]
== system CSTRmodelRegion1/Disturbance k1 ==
  Disturbance Change : Subsystem  Tag=STV Subsys  LoadFcn=sigbuilder_block('load');  StartFcn=sigbuilder_block('start');  StopFcn=sigbuilder_block('stop');  ClipboardFcn=sigbuilder_block('clipboard');
  Sum4 : Sum  Inputs=|++  OutDataType=fixdt(1, 16)  OutScaling=2^0
  Transfer Fcn (with initial outputs) : simulink_extras/Additional Linear/Transfer Fcn (with initial outputs)  SystemSampleTime=-1  N=[1]  D="[2  1]"  Y0=0  U0=0
  k1 : Step  Time=200  Before=0.3  After=0.3  SampleTime=0
  Out1 : Outport
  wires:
  k1/1 -> Sum4/1
  Sum4/1 -> Transfer Fcn (with initial outputs)/1
  Transfer Fcn (with initial outputs)/1 -> Out1/1
  Disturbance Change/1(Signal 1) -> Sum4/2

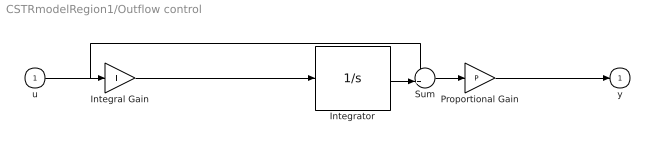
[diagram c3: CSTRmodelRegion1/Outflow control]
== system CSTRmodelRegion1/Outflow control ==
  u : Inport  OutDataType=OutDataTypeStr
  Integral Gain : Gain  DisableCoverage=on  Gain=I  ParamMin=IParamMin  ParamMax=IParamMax  ParameterDataTypeMode=Specify via dialog  ParameterDataType=IParamDataTypeStr  ParamDataTypeStr=IParamDataTypeStr  OutMin=IOutMin  OutMax=IOutMax  OutDataTypeMode=Specify via dialog  OutDataType=IOutDataTypeStr  OutDataTypeStr=IOutDataTypeStr
  Integrator : Integrator  DisableCoverage=on  InitialCondition=InitialConditionForIntegrator
  Proportional Gain : Gain  Gain=P  ParamMin=PParamMin  ParamMax=PParamMax  ParameterDataTypeMode=Specify via dialog  ParameterDataType=PParamDataTypeStr  ParamDataTypeStr=PParamDataTypeStr  OutMin=POutMin  OutMax=POutMax  OutDataTypeMode=Specify via dialog  OutDataType=POutDataTypeStr  OutDataTypeStr=POutDataTypeStr
  Sum : Sum  DisableCoverage=on  Inputs=++|  AccumDataTypeStr=SumAccumDataTypeStr  OutMin=SumOutMin  OutMax=SumOutMax  OutDataTypeMode=Specify via dialog  OutDataType=SumOutDataTypeStr  OutDataTypeStr=SumOutDataTypeStr
  y : Outport  OutDataType=OutDataTypeStr  InitialOutput=0
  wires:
  u/1 -> Sum/1, Integral Gain/1
  Proportional Gain/1 -> y/1
  Integral Gain/1 -> Integrator/1
  Integrator/1 -> Sum/2
  Sum/1 -> Proportional Gain/1

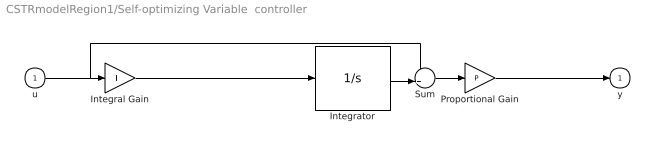
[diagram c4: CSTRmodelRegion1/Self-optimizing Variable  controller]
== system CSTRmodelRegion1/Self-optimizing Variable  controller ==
  u : Inport  OutDataType=OutDataTypeStr
  Integral Gain : Gain  DisableCoverage=on  Gain=I  ParamMin=IParamMin  ParamMax=IParamMax  ParameterDataTypeMode=Specify via dialog  ParameterDataType=IParamDataTypeStr  ParamDataTypeStr=IParamDataTypeStr  OutMin=IOutMin  OutMax=IOutMax  OutDataTypeMode=Specify via dialog  OutDataType=IOutDataTypeStr  OutDataTypeStr=IOutDataTypeStr
  Integrator : Integrator  DisableCoverage=on  InitialCondition=InitialConditionForIntegrator
  Proportional Gain : Gain  Gain=P  ParamMin=PParamMin  ParamMax=PParamMax  ParameterDataTypeMode=Specify via dialog  ParameterDataType=PParamDataTypeStr  ParamDataTypeStr=PParamDataTypeStr  OutMin=POutMin  OutMax=POutMax  OutDataTypeMode=Specify via dialog  OutDataType=POutDataTypeStr  OutDataTypeStr=POutDataTypeStr
  Sum : Sum  DisableCoverage=on  Inputs=++|  AccumDataTypeStr=SumAccumDataTypeStr  OutMin=SumOutMin  OutMax=SumOutMax  OutDataTypeMode=Specify via dialog  OutDataType=SumOutDataTypeStr  OutDataTypeStr=SumOutDataTypeStr
  y : Outport  OutDataType=OutDataTypeStr  InitialOutput=0
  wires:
  u/1 -> Sum/1, Integral Gain/1
  Proportional Gain/1 -> y/1
  Integral Gain/1 -> Integrator/1
  Integrator/1 -> Sum/2
  Sum/1 -> Proportional Gain/1

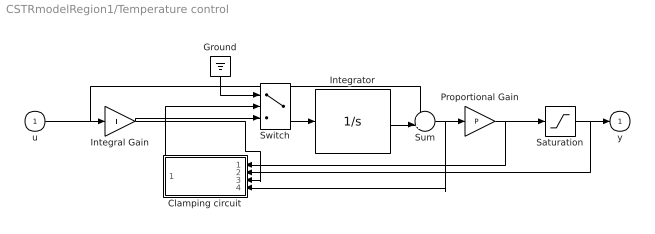
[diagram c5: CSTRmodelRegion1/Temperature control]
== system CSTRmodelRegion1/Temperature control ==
  u : Inport  OutDataType=OutDataTypeStr
  Clamping circuit : Subsystem
  Ground : Ground
  Integral Gain : Gain  DisableCoverage=on  Gain=I  ParamMin=IParamMin  ParamMax=IParamMax  ParameterDataTypeMode=Specify via dialog  ParameterDataType=IParamDataTypeStr  ParamDataTypeStr=IParamDataTypeStr  OutMin=IOutMin  OutMax=IOutMax  OutDataTypeMode=Specify via dialog  OutDataType=IOutDataTypeStr  OutDataTypeStr=IOutDataTypeStr
  Integrator : Integrator  DisableCoverage=on  InitialCondition=InitialConditionForIntegrator
  Proportional Gain : Gain  DisableCoverage=on  Gain=P  ParamMin=PParamMin  ParamMax=PParamMax  ParameterDataTypeMode=Specify via dialog  ParameterDataType=PParamDataTypeStr  ParamDataTypeStr=PParamDataTypeStr  OutMin=POutMin  OutMax=POutMax  OutDataTypeMode=Specify via dialog  OutDataType=POutDataTypeStr  OutDataTypeStr=POutDataTypeStr
  Saturation : Saturate  UpperLimit=UpperSaturationLimit  LowerLimit=LowerSaturationLimit  LinearizeAsGain=off  OutMin=SaturationOutMin  OutMax=SaturationOutMax  OutDataTypeMode=Specify via dialog  OutDataType=SaturationOutDataTypeStr  OutDataTypeStr=SaturationOutDataTypeStr
  Sum : Sum  DisableCoverage=on  Inputs=++|  AccumDataTypeStr=SumAccumDataTypeStr  OutMin=SumOutMin  OutMax=SumOutMax  OutDataTypeMode=Specify via dialog  OutDataType=SumOutDataTypeStr  OutDataTypeStr=SumOutDataTypeStr
  Switch : Switch  DisableCoverage=on  Criteria=u2 > Threshold
  y : Outport  OutDataType=OutDataTypeStr  InitialOutput=0
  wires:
  u/1 -> Sum/1, Integral Gain/1
  Integral Gain/1 -> Clamping circuit/3(preIntegrator), Switch/3
  Integrator/1 -> Sum/2
  Sum/1 -> Proportional Gain/1, Clamping circuit/4(preP)
  Saturation/1 -> y/1, Clamping circuit/2(postSat)
  Proportional Gain/1 -> Saturation/1, Clamping circuit/1(preSat)
  Ground/1 -> Switch/1
  Clamping circuit/1(Clamp) -> Switch/2
  Switch/1 -> Integrator/1

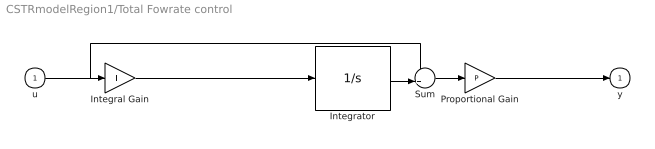
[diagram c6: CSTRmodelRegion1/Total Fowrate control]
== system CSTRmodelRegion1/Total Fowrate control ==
  u : Inport  OutDataType=OutDataTypeStr
  Integral Gain : Gain  DisableCoverage=on  Gain=I  ParamMin=IParamMin  ParamMax=IParamMax  ParameterDataTypeMode=Specify via dialog  ParameterDataType=IParamDataTypeStr  ParamDataTypeStr=IParamDataTypeStr  OutMin=IOutMin  OutMax=IOutMax  OutDataTypeMode=Specify via dialog  OutDataType=IOutDataTypeStr  OutDataTypeStr=IOutDataTypeStr
  Integrator : Integrator  DisableCoverage=on  InitialCondition=InitialConditionForIntegrator
  Proportional Gain : Gain  Gain=P  ParamMin=PParamMin  ParamMax=PParamMax  ParameterDataTypeMode=Specify via dialog  ParameterDataType=PParamDataTypeStr  ParamDataTypeStr=PParamDataTypeStr  OutMin=POutMin  OutMax=POutMax  OutDataTypeMode=Specify via dialog  OutDataType=POutDataTypeStr  OutDataTypeStr=POutDataTypeStr
  Sum : Sum  DisableCoverage=on  Inputs=++|  AccumDataTypeStr=SumAccumDataTypeStr  OutMin=SumOutMin  OutMax=SumOutMax  OutDataTypeMode=Specify via dialog  OutDataType=SumOutDataTypeStr  OutDataTypeStr=SumOutDataTypeStr
  y : Outport  OutDataType=OutDataTypeStr  InitialOutput=0
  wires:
  u/1 -> Sum/1, Integral Gain/1
  Proportional Gain/1 -> y/1
  Integral Gain/1 -> Integrator/1
  Integrator/1 -> Sum/2
  Sum/1 -> Proportional Gain/1

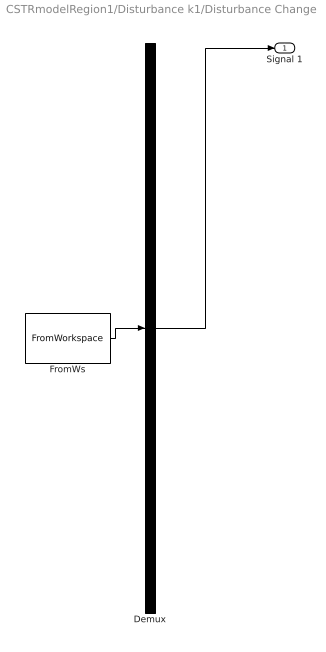
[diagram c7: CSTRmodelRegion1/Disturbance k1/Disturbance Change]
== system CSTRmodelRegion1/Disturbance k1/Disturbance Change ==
  Demux : Demux  Tag=STV Demux  Outputs=1
  FromWs : FromWorkspace  Tag=STV FromWs  VariableName=tuvar  SampleTime=0  SigBuilderData=DataTag0  VnvData=DataTag1
  Signal 1 : Outport  Tag=STV Outport  OutDataType=fixdt(1, 16)  OutScaling=2^0
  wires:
  FromWs/1 -> Demux/1
  Demux/1 -> Signal 1/1

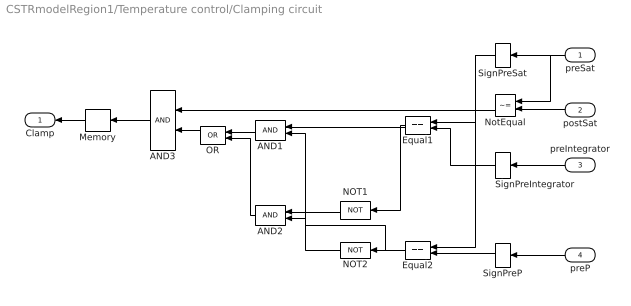
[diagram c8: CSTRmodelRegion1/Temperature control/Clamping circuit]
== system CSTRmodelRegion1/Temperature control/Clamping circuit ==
  preSat : Inport
  postSat : Inport  Port=2
  preIntegrator : Inport  Port=3
  preP : Inport  Port=4
  AND1 : Logic  DisableCoverage=on  OutDataTypeMode=boolean  OutDataTypeStr=boolean
  AND2 : Logic  DisableCoverage=on  OutDataTypeMode=boolean  OutDataTypeStr=boolean
  AND3 : Logic  DisableCoverage=on  OutDataTypeMode=boolean  OutDataTypeStr=boolean
  Equal1 : RelationalOperator  DisableCoverage=on  Operator===  LogicOutDataTypeMode=boolean  OutDataTypeStr=boolean
  Equal2 : RelationalOperator  DisableCoverage=on  Operator===  LogicOutDataTypeMode=boolean  OutDataTypeStr=boolean
  Memory : Memory
  NOT1 : Logic  DisableCoverage=on  Operator=NOT  OutDataTypeMode=boolean  OutDataTypeStr=boolean
  NOT2 : Logic  DisableCoverage=on  Operator=NOT  OutDataTypeMode=boolean  OutDataTypeStr=boolean
  NotEqual : RelationalOperator  DisableCoverage=on  Operator=~=  LogicOutDataTypeMode=boolean  OutDataTypeStr=boolean
  OR : Logic  DisableCoverage=on  Operator=OR  OutDataTypeMode=boolean  OutDataTypeStr=boolean
  SignPreIntegrator : Signum  DisableCoverage=on
  SignPreP : Signum  DisableCoverage=on
  SignPreSat : Signum  DisableCoverage=on
  Clamp : Outport
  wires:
  preSat/1 -> SignPreSat/1, NotEqual/1
  postSat/1 -> NotEqual/2
  preIntegrator/1 -> SignPreIntegrator/1
  preP/1 -> SignPreP/1
  SignPreSat/1 -> Equal1/1, Equal2/1
  NotEqual/1 -> AND3/1
  SignPreIntegrator/1 -> Equal1/2
  SignPreP/1 -> Equal2/2
  Equal1/1 -> AND1/1, NOT1/1
  Equal2/1 -> AND1/2, NOT2/1
  NOT1/1 -> AND2/1
  NOT2/1 -> AND2/2
  AND1/1 -> OR/1
  AND2/1 -> OR/2
  OR/1 -> AND3/2
  AND3/1 -> Memory/1
  Memory/1 -> Clamp/1

== matlab function Self-optimizing 
Variable ==
function cs = fcn(Fa,Fb,V,cVector)


cain        =  2;
cbin        = 1.5;
Fmax        = 22;
k2          =  0.0140;
cb          =  cVector(2);

%cs = (-cbin^2*Fa^2-Fa^2*cain*cbin+6*Fa*cain*k2*cb^2*V+2*Fa*cain*Fmax*cb-Fa*cain*Fmax*cbin+4*V*k2*cb^3*Fmax+4*V^2*k2^2*cb^4-2*cbin*Fmax^2*cb+Fmax^2*cb^2-4*V*k2*cb^2*cbin*Fmax+cbin^2*Fmax^2)/Fmax;
%cs =cs/V;
cs = (-cbin^2*Fa^2-Fa^2*cain*cbin+6*Fa*cain*k2*cb^2*V+2*Fa*cain*Fmax*cb-Fa*cain*Fmax*cbin+4*V*k2*cb^3*Fmax+4*V^2*k2^2*cb^4-2*cbin*Fmax^2*cb+Fmax^2*cb^2-4*V*k2*cb^2*cbin*Fmax+cbin^2*Fmax^2);
%cs =cs/V;

== matlab function Self-optimizing 
Variable Region 3 ==
function cs = SOCVariable3(Fa,Fb,V,cVector)


cain        =  2;
cbin        = 1.5;
Fmax        = 22;
k2          =  0.0140;
cb          =  cVector(2);
H1          = -70;
H2          = -50;
qmax        = 1e3;



ScaleFactor = 2.5;

cs = (-4*V*cb^2*k2*H2*Fa*cain*cbin*qmax*H1+Fa*cbin^2*qmax^2*H1+4*V^2*cb^4*k2^2*H2*Fa*cain*cbin*H1^2-4*V^2*cb^4*k2^2*H2^2*Fa*cain*cbin*H1-2*V*cb^2*k2*Fa*cain*cbin*H1^2*qmax-4*V*cb^2*k2*H2*Fa*cbin^2*H1*qmax-2*V*cb^2*k2*H2*Fa^2*cain*cbin^2*H1^2+8*V*cb^3*k2*H2*H1*Fa*cain*qmax-8*V^2*cb^4*k2^2*H2*cbin*H1*qmax-12*V^2*cb^4*k2^2*Fa*H2^2*cbin^2*H1-8*V^2*cb^5*k2^2*H2*Fa*cain*H1^2+8*V^2*cb^5*k2^2*H2^2*H1*Fa*cain+8*V^2*cb^5*k2^2*Fa*H2^2*cbin*H1-qmax^3*cbin+2*cb*qmax^3-H1*cbin*Fa*cain*qmax^2+2*cb*Fa*cain*qmax^2*H1+Fa^2*cain*cbin^2*H1^2*qmax-2*cb*Fa*cbin*qmax^2*H1+8*V*cb^3*k2*H2*qmax^2+8*V^2*cb^5*k2^2*H2^2*qmax+8*V^3*cb^6*k2^3*H2^3*cbin-2*cb*Fa^2*cain*cbin*H1^2*qmax-2*V*cb^2*k2*H1*qmax^2*cbin-2*V*cb^2*k2*H2*qmax^2*cbin+4*V^2*cb^4*k2^2*H2^2*cbin*qmax-8*V^3*cb^6*k2^3*H2^2*cbin*H1)/(H1^2*H2*Fa*Fb); %*1.2250e-19;
cs=cs/ScaleFactor;
